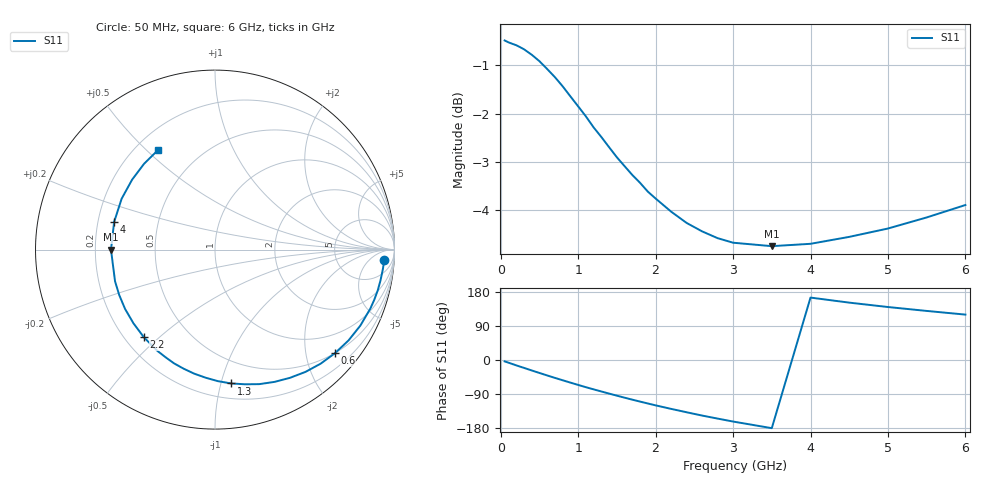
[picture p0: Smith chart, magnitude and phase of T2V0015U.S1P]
! SIEMENS Discrete & RF Semiconductors
! BAS70-04W
! Si Schottky Diode in SOT323
! IF = 0.015 mA
! S-Parameters:  November  1997
# GHz  S  MA  R  50
!  f  S11
! GHz  MAG  ANG
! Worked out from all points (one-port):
!   34 points, 50 MHz to 6 GHz, reference 50 ohm
!   lowest |S11| = -4.7 dB at 3.5 GHz (marker M1), VSWR 3.76, Z = 13.3 - j0.0405 ohm
!   |S11| at or under -10 dB: nowhere
!   S11 on the Smith chart (normalised r, x): 50 MHz: 16, -18; 600 MHz: 0.50, -2.61; 1.3 GHz: 0.31, -1.08; 2.2 GHz: 0.28, -0.45; 4 GHz: 0.27, +0.12; 6 GHz: 0.29, +0.54
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0.05  0.9454 -3.6
0.2  0.9347 -14.1
0.3  0.9257 -20.8
0.4  0.9138 -27.6
0.5  0.8998 -34.2
0.6  0.8832 -40.8
0.7  0.8662 -47.2
0.8  0.8476 -53.5
0.9  0.8275 -59.7
1  0.8081 -65.8
1.1  0.789 -71.8
1.3  0.7512 -83.1
1.4  0.7332 -88.7
1.6  0.7009 -99.5
1.8  0.6736 -109.8
1.9  0.6597 -114.8
2  0.649 -119.7
2.2  0.6291 -129.0
2.4  0.6124 -137.9
2.6  0.6002 -146.6
2.8  0.5906 -154.6
3  0.5843 -162.4
3.5  0.5795 -179.9
4  0.5827 164.7
4.5  0.5924 151.4
5  0.6043 139.8
5.5  0.6205 129.5
6  0.6391 119.8
